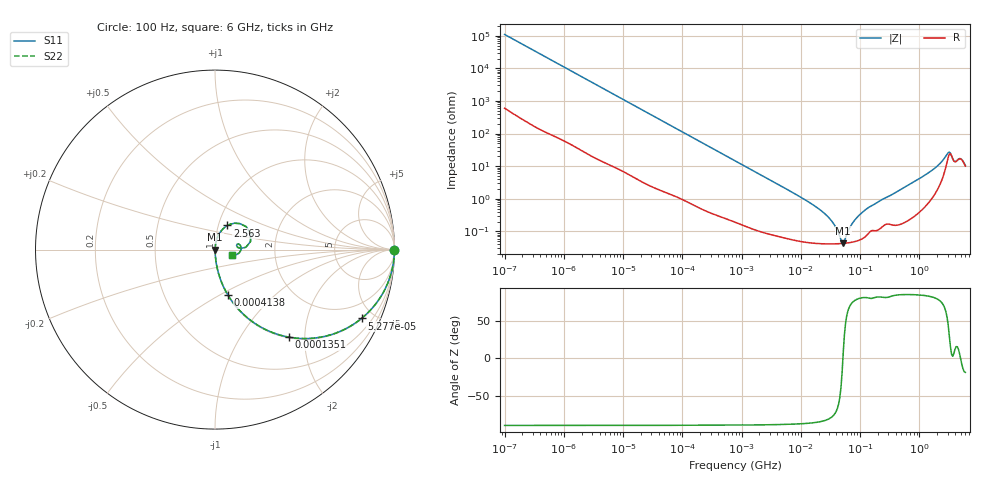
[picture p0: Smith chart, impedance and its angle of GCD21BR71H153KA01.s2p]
!Murata Part Number: GCD21BR71H153KA01
!These Parameters are Measured in Series Mode Connection
!Data Generated on Jan 08, 2026
!  o--ll--o
!Port1  Port2
!  o------o
!Operation Temp=25[degC], DC Bias Voltage=0[V]
!Freq. Start=100[Hz] Stop=6[GHz] 401[Steps]
# Hz S RI R 50
!Freq.(Hz) S11(Real) S11(Imag) S21(Real) S21(Imag) S12(Real) S12(Imag) S22(Real) S22(Imag)
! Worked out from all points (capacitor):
!   401 points, 100 Hz to 6 GHz, reference 50 ohm
!   read as one part in series: C = 14.5 nF near 109 Hz
!   lowest |Z| = 43.3 mohm at 52.11 MHz (marker M1)
!   series resonance near 51.39 MHz, so ESL is about 660 pH
!   S11 on the Smith chart (normalised r, x): 100 Hz: open; 52.77 kHz: 1.03, -4.24; 135.1 kHz: 1.01, -1.66; 413.8 kHz: 1.01, -0.55; 2.563 GHz: 1.11, +0.30; 6 GHz: 1.20, -0.07
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100  1 -0.000913  5.8e-06 0.000913  5.8e-06 0.000913  1 -0.000913
2008  0.9996 -0.0182  0.000428 0.0182  0.000428 0.0182  0.9996 -0.0182
11514  0.9888 -0.1022  0.0112 0.1022  0.0112 0.1022  0.9888 -0.1022
40335  0.8831 -0.3179  0.1169 0.3179  0.1169 0.3179  0.8831 -0.3179
52766  0.8163 -0.3836  0.1837 0.3836  0.1837 0.3836  0.8163 -0.3836
135116  0.41 -0.4875  0.59 0.4875  0.59 0.4875  0.41 -0.4875
413847  0.0718 -0.2529  0.9282 0.2529  0.9282 0.2529  0.0718 -0.2529
774597  0.0228 -0.143  0.9772 0.143  0.9772 0.143  0.0228 -0.143
1.555665e7  0.000483 -0.00677  0.9995 0.00677  0.9995 0.00677  0.000483 -0.00677
3.184506e7  0.000418 -0.00225  0.9996 0.00225  0.9996 0.00225  0.000418 -0.00225
3.80911e7  0.000417 -0.00138  0.9996 0.00138  0.9996 0.00138  0.000417 -0.00138
4.764863e7  0.000423 -0.000342  0.9996 0.000342  0.9996 0.000342  0.000423 -0.000342
5.211241e7  0.000428 6.45e-05  0.9996 -6.45e-05  0.9996 -6.45e-05  0.000428 6.45e-05
7.129496e7  0.000464 0.00152  0.9995 -0.00152  0.9995 -0.00152  0.000464 0.00152
9.753859e7  0.000549 0.00313  0.9995 -0.00313  0.9995 -0.00313  0.000549 0.00313
3.124326e8  0.0018 0.012  0.9982 -0.012  0.9982 -0.012  0.0018 0.012
1.369159e9  0.0102 0.0581  0.9898 -0.0581  0.9898 -0.0581  0.0102 0.0581
2.562649e9  0.0694 0.1343  0.9306 -0.1343  0.9306 -0.1343  0.0694 0.1343
3.205649e9  0.1987 0.0911  0.8013 -0.0911  0.8013 -0.0911  0.1987 0.0911
4.009986e9  0.12 0.0226  0.88 -0.0226  0.88 -0.0226  0.12 0.0226
5.016141e9  0.1443 -0.00314  0.8557 0.00314  0.8557 0.00314  0.1443 -0.00314
6e9  0.0923 -0.0282  0.9077 0.0282  0.9077 0.0282  0.0923 -0.0282
